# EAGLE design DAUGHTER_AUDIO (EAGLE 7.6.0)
DAUGHTER CARD AUDIO

## Sheet 1 of 3: HDK INTERFACE
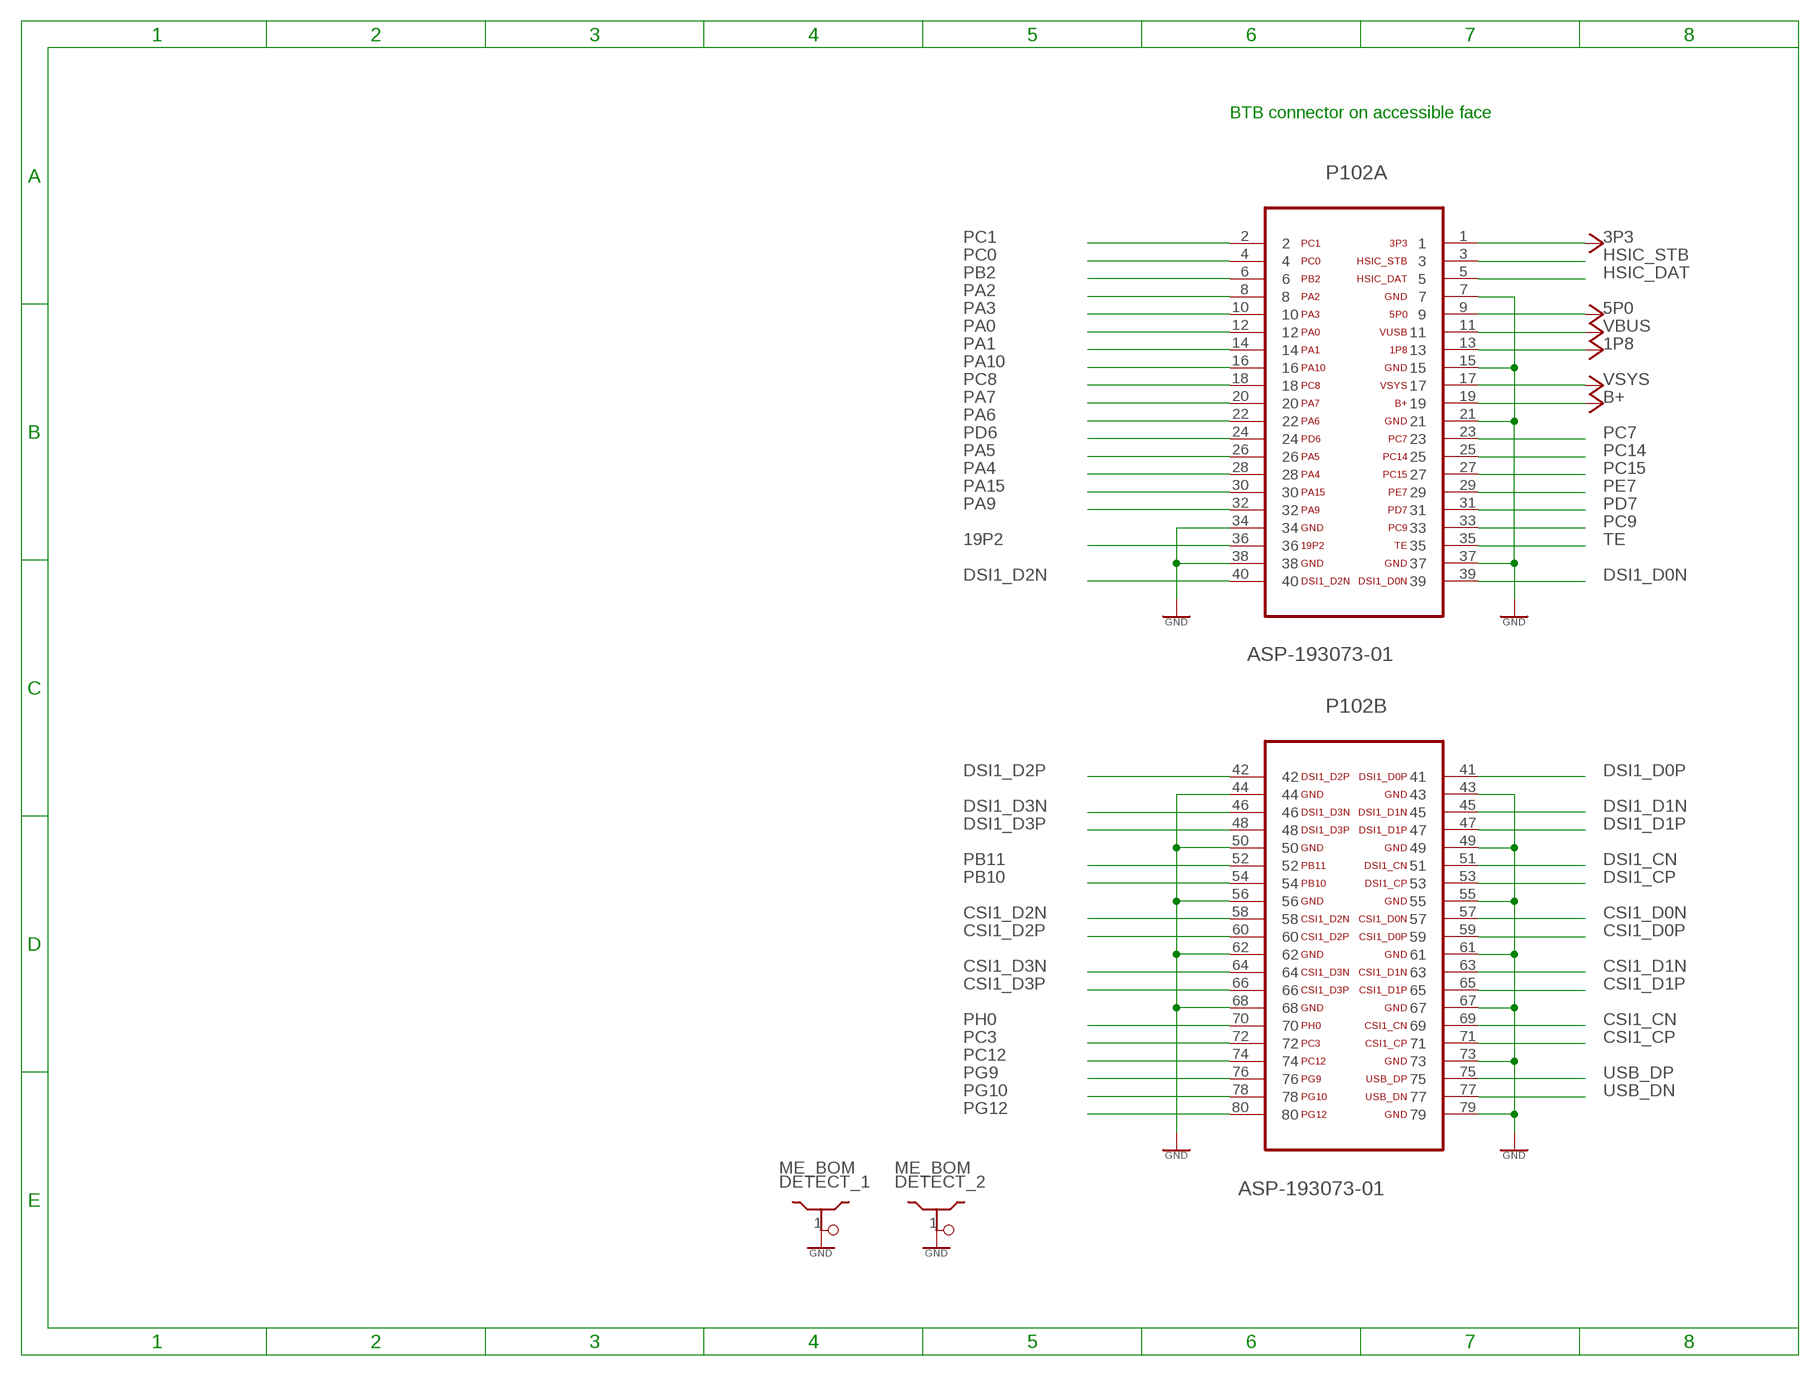
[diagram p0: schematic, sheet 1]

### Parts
DETECT_1  ME_BOM  SHIELDDETECT  [PLUG]
DETECT_2  ME_BOM  SHIELDDETECT  [PLUG]
P102  ASP-193073-01  FTMH-140-02-L-DV-ES-P-TR  [FTMH-140-02-L-DV-ES-P-TR]

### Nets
1P8: P102.13 ; also sheet 2,3
3P3: P102.1 ; also sheet 2
5P0: P102.9
19P2: P102.36
B+: P102.19 ; also sheet 3
CSI1_CN: P102.69
CSI1_CP: P102.71
CSI1_D0N: P102.57
CSI1_D0P: P102.59
CSI1_D1N: P102.63
CSI1_D1P: P102.65
CSI1_D2N: P102.58
CSI1_D2P: P102.60
CSI1_D3N: P102.64
CSI1_D3P: P102.66
DSI1_CN: P102.51
DSI1_CP: P102.53
DSI1_D0N: P102.39
DSI1_D0P: P102.41
DSI1_D1N: P102.45
DSI1_D1P: P102.47
DSI1_D2N: P102.40
DSI1_D2P: P102.42
DSI1_D3N: P102.46
DSI1_D3P: P102.48
GND: DETECT_1.1 DETECT_2.1 P102.7 P102.15 P102.21 P102.34 P102.37 P102.38 P102.43 P102.44 P102.49 P102.50 P102.55 P102.56 P102.61 P102.62 P102.67 P102.68 P102.73 P102.79 ; also sheet 2,3
HSIC_DAT: P102.5
HSIC_STB: P102.3
PA0: P102.12
PA1: P102.14
PA2: P102.8
PA3: P102.10
PA4: P102.28
PA5: P102.26
PA6: P102.22
PA7: P102.20
PA9: P102.32
PA10: P102.16
PA15: P102.30
PB2: P102.6
PB10: P102.54 ; also sheet 2
PB11: P102.52 ; also sheet 2
PC0: P102.4 ; also sheet 3
PC1: P102.2 ; also sheet 3
PC3: P102.72
PC7: P102.23 ; also sheet 3
PC8: P102.18
PC9: P102.33
PC12: P102.74
PC14: P102.25 ; also sheet 3
PC15: P102.27 ; also sheet 3
PD6: P102.24
PD7: P102.31 ; also sheet 3
PE7: P102.29 ; also sheet 3
PG9: P102.76 ; also sheet 2
PG10: P102.78 ; also sheet 3
PG12: P102.80
PH0: P102.70 ; also sheet 3
TE: P102.35
USB_DN: P102.77
USB_DP: P102.75
VBUS: P102.11
VSYS: P102.17

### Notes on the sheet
- BTB connector on accessible face

## Sheet 2 of 3: Identification
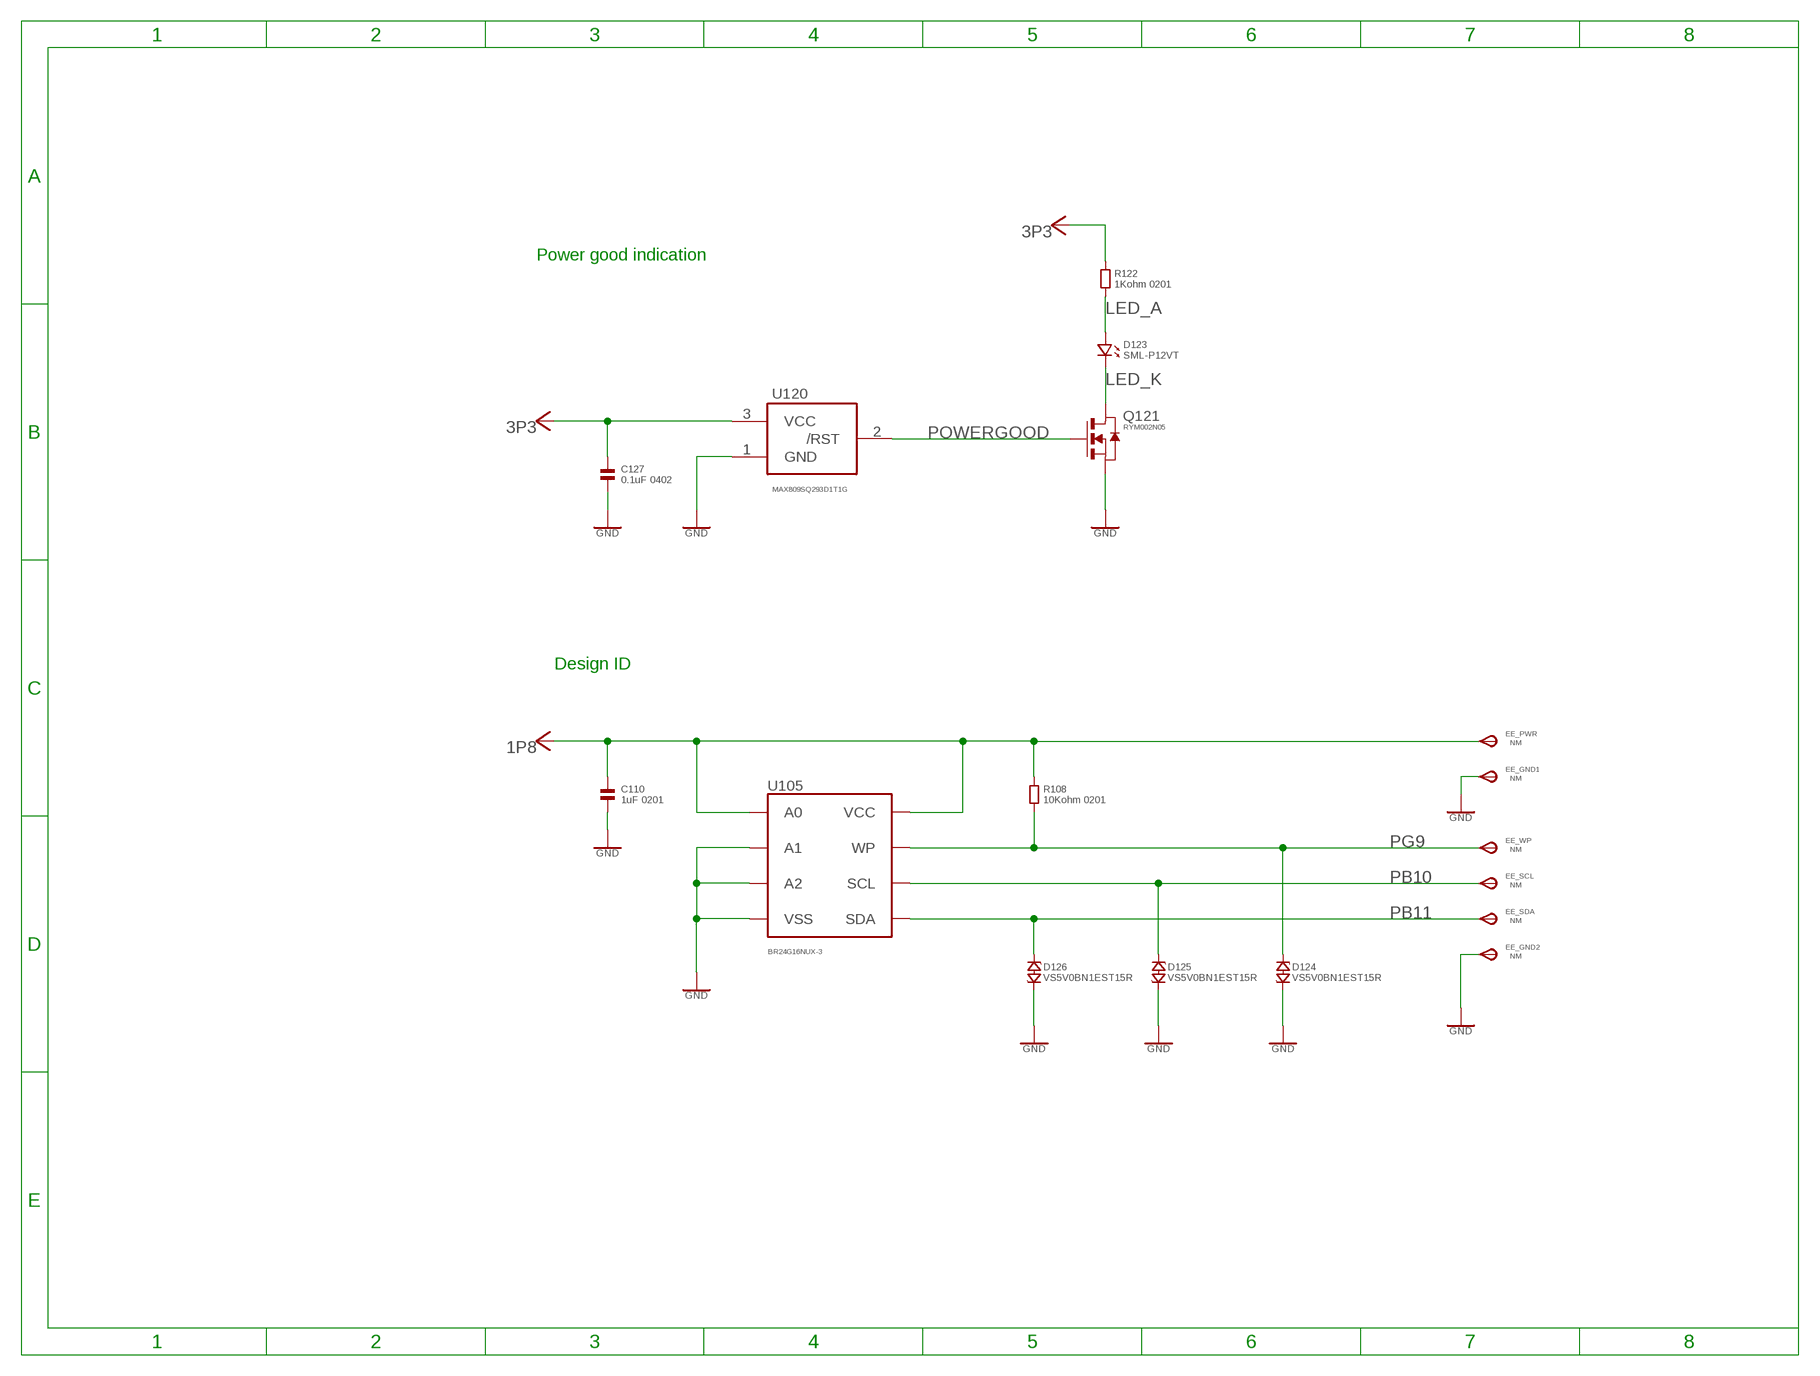
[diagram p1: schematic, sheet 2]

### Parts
C110  1uF 0201  CAPACITOR.0201  [0201]
C127  0.1uF 0402  CAPACITOR.0402  [0402]
D123  SML-P12VT  LED.0503  [0503.LED]
D124  VS5V0BN1EST15R  ESD_VARISTOR.0201  [CHIP_0201]
D125  VS5V0BN1EST15R  ESD_VARISTOR.0201  [CHIP_0201]
D126  VS5V0BN1EST15R  ESD_VARISTOR.0201  [CHIP_0201]
EE_GND1  NM  TPSTP11R  [TP11R]
EE_GND2  NM  TPSTP11R  [TP11R]
EE_PWR  NM  TPSTP11R  [TP11R]
EE_SCL  NM  TPSTP11R  [TP11R]
EE_SDA  NM  TPSTP11R  [TP11R]
EE_WP  NM  TPSTP11R  [TP11R]
Q121  RYM002N05  FET-NRYM002N05  [VMT3]
R108  10Kohm 0201  RESISTOR.0201  [0201]
R122  1Kohm 0201  RESISTOR.0201  [0201]
U105  BR24G16NUX-3  EEPROMDFN8  [DFN-8]
U120  MAX809SQ293D1T1G  MAX809  [SC70-3L]

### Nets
1P8: C110.1 EE_PWR.TP(PP) R108.1 U105.P$1(A0) U105.P$8(VCC) ; also sheet 1,3
3P3: C127.1 R122.1 U120.3(VCC) ; also sheet 1
GND: C110.2 C127.2 D124.P$2 D125.P$2 D126.P$2 EE_GND1.TP(PP) EE_GND2.TP(PP) Q121.2(S) U105.P$2(A1) U105.P$3(A2) U105.P$4(VSS) U105.P$9(VSS) U120.1(GND) ; also sheet 1,3
LED_A: D123.P$1 R122.2
LED_K: D123.P$2 Q121.3(D)
PB10: D125.P$1 EE_SCL.TP(PP) U105.P$6(SCL) ; also sheet 1
PB11: D126.P$1 EE_SDA.TP(PP) U105.P$5(SDA) ; also sheet 1
PG9: D124.P$1 EE_WP.TP(PP) R108.2 U105.P$7(WP) ; also sheet 1
POWERGOOD: Q121.1(G) U120.2(/RST)

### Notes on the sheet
- Power good indication
- Design ID

## Sheet 3 of 3: LOUD SPEAKER
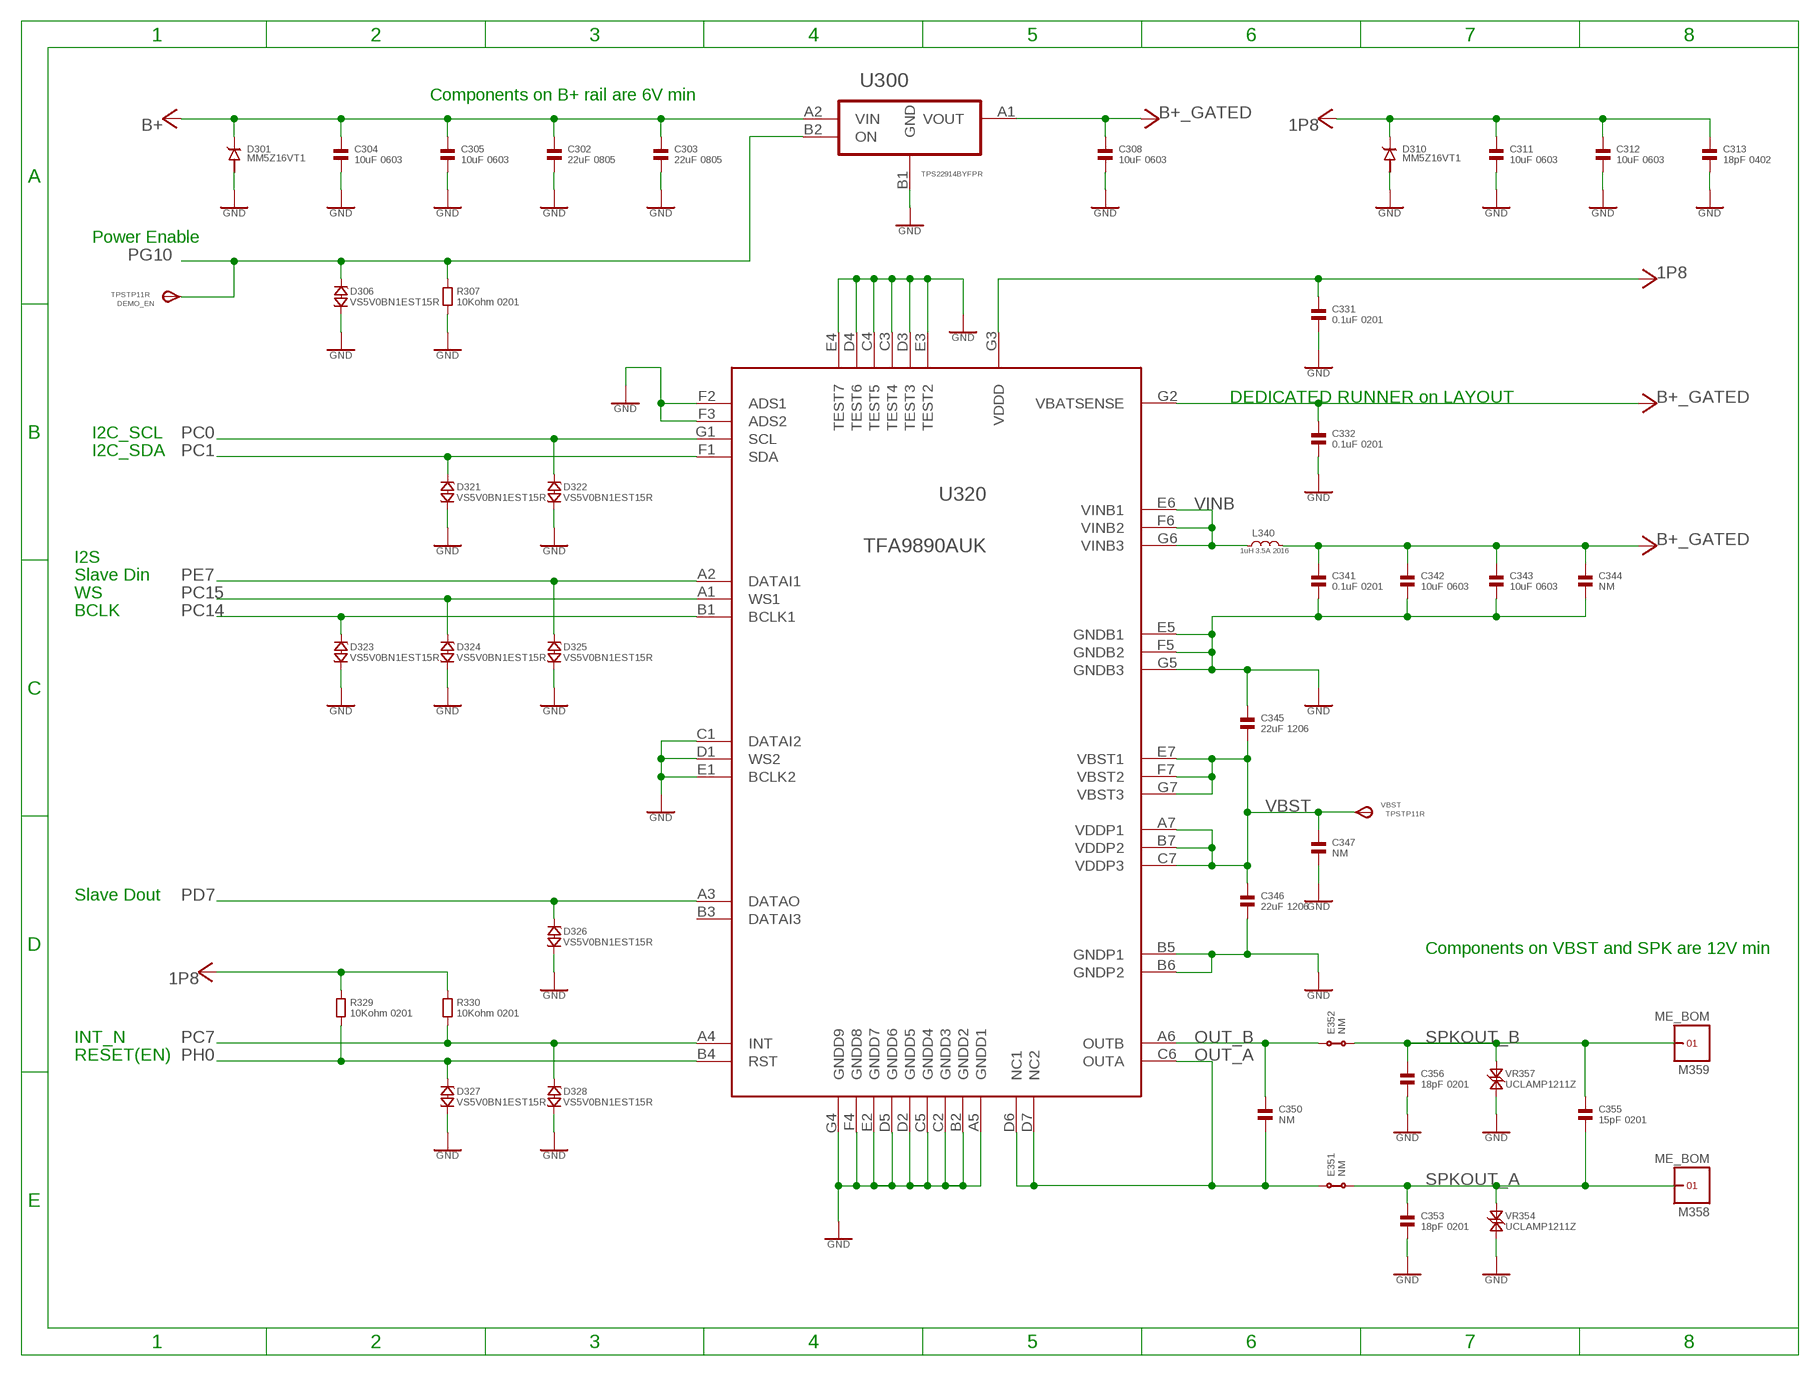
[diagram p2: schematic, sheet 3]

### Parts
C302  22uF 0805  CAPACITOR.0805  [0805]
C303  22uF 0805  CAPACITOR.0805  [0805]
C304  10uF 0603  CAPACITOR.0603  [0603]
C305  10uF 0603  CAPACITOR.0603  [0603]
C308  10uF 0603  CAPACITOR.0603  [0603]
C311  10uF 0603  CAPACITOR.0603  [0603]
C312  10uF 0603  CAPACITOR.0603  [0603]
C313  18pF 0402  CAPACITOR.0402  [0402]
C331  0.1uF 0201  CAPACITOR.0201  [0201]
C332  0.1uF 0201  CAPACITOR.0201  [0201]
C341  0.1uF 0201  CAPACITOR.0201  [0201]
C342  10uF 0603  CAPACITOR.0603  [0603]
C343  10uF 0603  CAPACITOR.0603  [0603]
C344  NM  CAPACITOR.0402  [0402]
C345  22uF 1206  CAPACITOR.1206  [1206]
C346  22uF 1206  CAPACITOR.1206  [1206]
C347  NM  CAPACITOR.0402  [0402]
C350  NM  CAPACITOR.0201  [0201]
C353  18pF 0201  CAPACITOR.0201  [0201]
C355  15pF 0201  CAPACITOR.0201  [0201]
C356  18pF 0201  CAPACITOR.0201  [0201]
D301  MM5Z16VT1  DIODE.SOD523  [SOD523]
D306  VS5V0BN1EST15R  ESD_VARISTOR.0201  [CHIP_0201]
D310  MM5Z16VT1  DIODE.SOD523  [SOD523]
D321  VS5V0BN1EST15R  ESD_VARISTOR.0201  [CHIP_0201]
D322  VS5V0BN1EST15R  ESD_VARISTOR.0201  [CHIP_0201]
D323  VS5V0BN1EST15R  ESD_VARISTOR.0201  [CHIP_0201]
D324  VS5V0BN1EST15R  ESD_VARISTOR.0201  [CHIP_0201]
D325  VS5V0BN1EST15R  ESD_VARISTOR.0201  [CHIP_0201]
D326  VS5V0BN1EST15R  ESD_VARISTOR.0201  [CHIP_0201]
D327  VS5V0BN1EST15R  ESD_VARISTOR.0201  [CHIP_0201]
D328  VS5V0BN1EST15R  ESD_VARISTOR.0201  [CHIP_0201]
DEMO_EN  TPSTP11R  [TP11R]
E351  NM  SHORT_BAR.0603  [0603_SHORT]
E352  NM  SHORT_BAR.0603  [0603_SHORT]
L340  1uH 3.5A 2016  POWER-INDUCTOR.2016  [2016]
M358  ME_BOM  PUCK.PUCK  [PUCK]
M359  ME_BOM  PUCK.PUCK  [PUCK]
R307  10Kohm 0201  RESISTOR.0201  [0201]
R329  10Kohm 0201  RESISTOR.0201  [0201]
R330  10Kohm 0201  RESISTOR.0201  [0201]
U300  TPS22914BYFPR  [BGA0_75SQ_PS0_4_P4]
U320  TFA9890AUK  [BGA7X7]
VBST  TPSTP11R  [TP11R]
VR354  UCLAMP1211Z  ESD_TVS.0201  [CHIP_0201]
VR357  UCLAMP1211Z  ESD_TVS.0201  [CHIP_0201]

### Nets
1P8: C311.1 C312.1 C313.1 C331.1 D310.1 R329.1 R330.1 U320.G3(VDDD) ; also sheet 1,2
B+: C302.1 C303.1 C304.1 C305.1 D301.1 U300.A2(VIN) ; also sheet 1
B+_GATED: C308.1 C332.1 C341.1 C342.1 C343.1 C344.1 L340.2 U300.A1(VOUT) U320.G2(VBATSENSE)
GND: C302.2 C303.2 C304.2 C305.2 C308.2 C311.2 C312.2 C313.2 C331.2 C332.2 C341.2 C342.2 C343.2 C344.2 C345.1 C346.2 C347.2 C353.2 C356.2 D301.2 D306.P$2 D310.2 D321.P$2 D322.P$2 D323.P$2 D324.P$2 D325.P$2 D326.P$2 D327.P$2 D328.P$2 R307.2 U300.B1(GND) U320.A5(GNDD1) U320.B2(GNDD2) U320.B5(GNDP1) U320.B6(GNDP2) U320.C1(DATAI2) U320.C2(GNDD3) U320.C3(TEST4) U320.C4(TEST5) U320.C5(GNDD4) U320.D1(WS2) U320.D2(GNDD5) U320.D3(TEST3) U320.D4(TEST6) U320.D5(GNDD6) U320.E1(BCLK2) U320.E2(GNDD7) U320.E3(TEST2) U320.E4(TEST7) U320.E5(GNDB1) U320.F2(ADS1) U320.F3(ADS2) U320.F4(GNDD8) U320.F5(GNDB2) U320.G4(GNDD9) U320.G5(GNDB3) VR354.P$2 VR357.P$2 ; also sheet 1,2
OUT_A: C350.2 E351.1 U320.C6(OUTA) U320.D6(NC1) U320.D7(NC2)
OUT_B: C350.1 E352.1 U320.A6(OUTB)
PC0: D322.P$1 U320.G1(SCL) ; also sheet 1
PC1: D321.P$1 U320.F1(SDA) ; also sheet 1
PC7: D328.P$1 R330.2 U320.A4(INT) ; also sheet 1
PC14: D323.P$1 U320.B1(BCLK1) ; also sheet 1
PC15: D324.P$1 U320.A1(WS1) ; also sheet 1
PD7: D326.P$1 U320.A3(DATAO) ; also sheet 1
PE7: D325.P$1 U320.A2(DATAI1) ; also sheet 1
PG10: D306.P$1 DEMO_EN.TP(PP) R307.1 U300.B2(ON) ; also sheet 1
PH0: D327.P$1 R329.2 U320.B4(RST) ; also sheet 1
SPKOUT_A: C353.1 C355.2 E351.2 M358.1 VR354.P$1
SPKOUT_B: C355.1 C356.1 E352.2 M359.1 VR357.P$1
VBST: C345.2 C346.1 C347.1 U320.A7(VDDP1) U320.B7(VDDP2) U320.C7(VDDP3) U320.E7(VBST1) U320.F7(VBST2) U320.G7(VBST3) VBST.TP(PP)
VINB: L340.1 U320.E6(VINB1) U320.F6(VINB2) U320.G6(VINB3)
Unconnected: U320.B3(DATAI3)

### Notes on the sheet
- Components on B+ rail are 6V min
- Power Enable
- DEDICATED RUNNER on LAYOUT
- I2C_SCL
- I2C_SDA
- I2S
- Slave Din
- WS
- BCLK
- Slave Dout
- Components on VBST and SPK are 12V min
- INT_N
- RESET(EN)

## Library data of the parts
C110 C127 C302-C305 C308 C311-C313 C331 C332 C341-C347 C350 C353 C355 C356 = MOTO_LIB:CAPACITOR: Ceramic Capacitor, Generic
D123 = MOTO_LIB:LED: LED GENERIC, single, 2 pin; MPN: SML-P12VT; SUPPLIER: ROHM
D124-D126 D306 D321-D328 = MOTO_LIB:ESD_VARISTOR: GENERIC varistor,single, 2 pin; MPN: VS5V0BN1EST15R; SUPPLIER: ROHM
D301 D310 = MOTO_LIB:DIODE: DIODE GENERIC, single, 2 pin; MPN: MM5Z16VT1; SUPPLIER: ON_SEMI
DEMO_EN EE_GND1 EE_GND2 EE_PWR EE_SCL EE_SDA EE_WP VBST = MOTO_LIB:TPS: TEST Point, 1mm diameter, gold
DETECT_1 DETECT_2 = MOTO_LIB:SHIELD: Shield, Custom; MPN: refer to ME BOM; SUPPLIER: ref to ME BOM
E351 E352 = MOTO_LIB:SHORT_BAR: SHORT BAR - layout feature
L340 = MOTO_LIB:POWER-INDUCTOR: Inductor, Power
M358 M359 = MOTO_LIB:PUCK: test pad; MPN: refer to ME BOM; SUPPLIER: refer to ME BOM
P102 = MOTO_LIB:FTMH-140-02-L-DV-ES-P-TR: MICRO SOCKET, 1.0MM, SMD, 2X40WAY, MALE; MPN: ASP-193073-01; SUPPLIER: SAMTEC
Q121 = MOTO_LIB:FET-N: Generic NMOS FET; MPN: RYM002N05; SUPPLIER: ROHM
R108 R122 R307 R329 R330 = MOTO_LIB:RESISTOR: Resistor - Generic
U105 = MOTO_LIB:EEPROM: I2C EE PROM, 8 pin; MPN: BR24G16NUX-3; SUPPLIER: ROHM
U120 = MOTO_LIB:MAX809: 3-Pin Microprocessor Reset Circuit; MPN: MAX809SQ293D1T1; SUPPLIER: ON-SEMI
U300 = MOTO_LIB:TPS22914BYFPR: 5V load switch; MPN: TPS22914BYFPR; SUPPLIER: TI
U320 = MOTO_LIB:TFA9890AUK: Audio Power amplifier; MPN: TFA9890AUK; SUPPLIER: NXP
VR354 VR357 = MOTO_LIB:ESD_TVS: GENERIC TVS,single, 2 pin; MPN: UCLAMP1211Z; SUPPLIER: SEMTECH

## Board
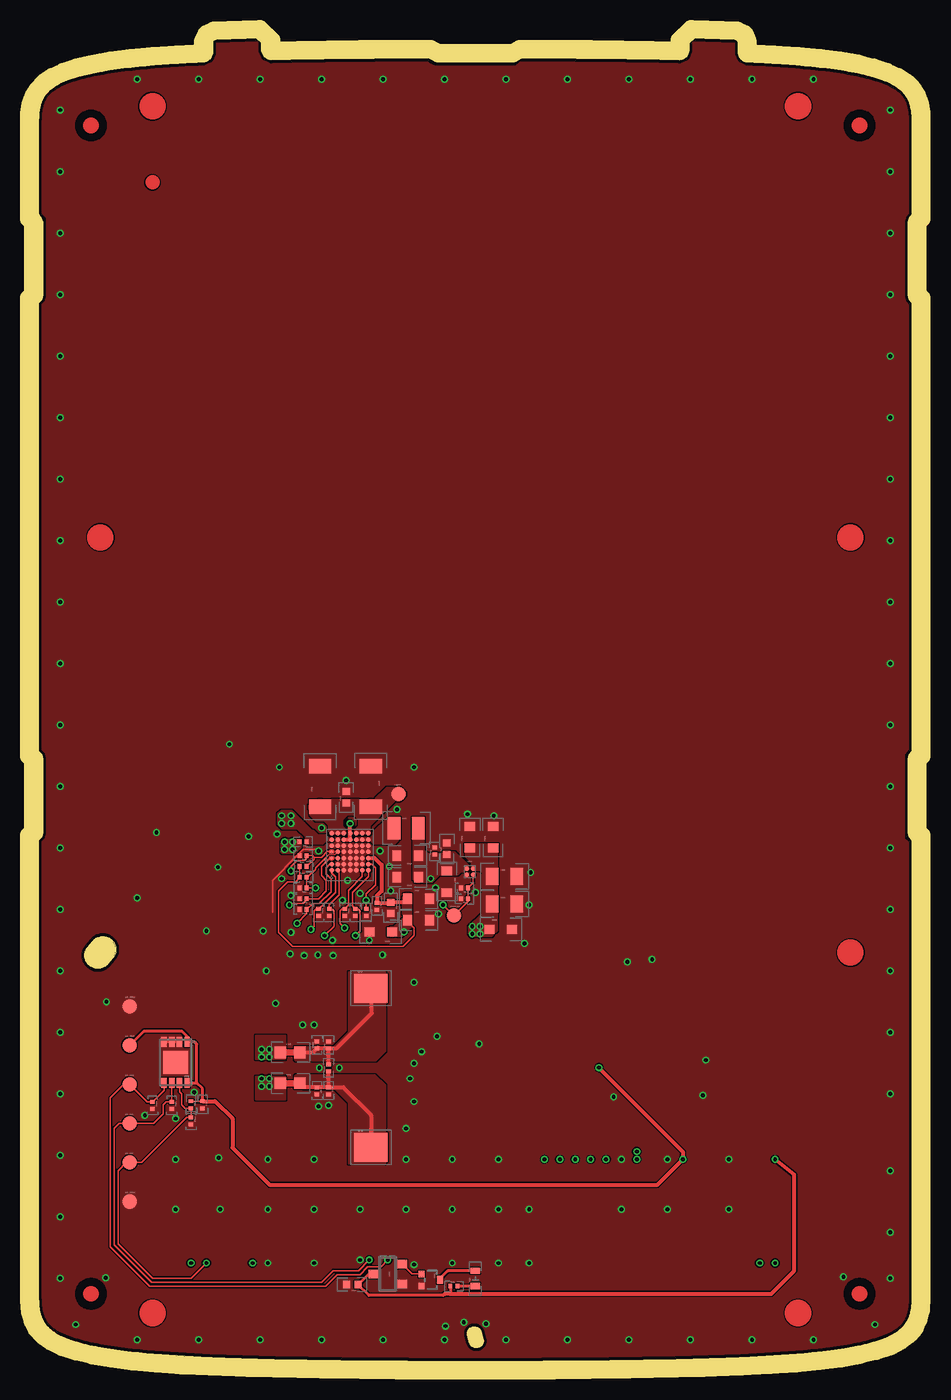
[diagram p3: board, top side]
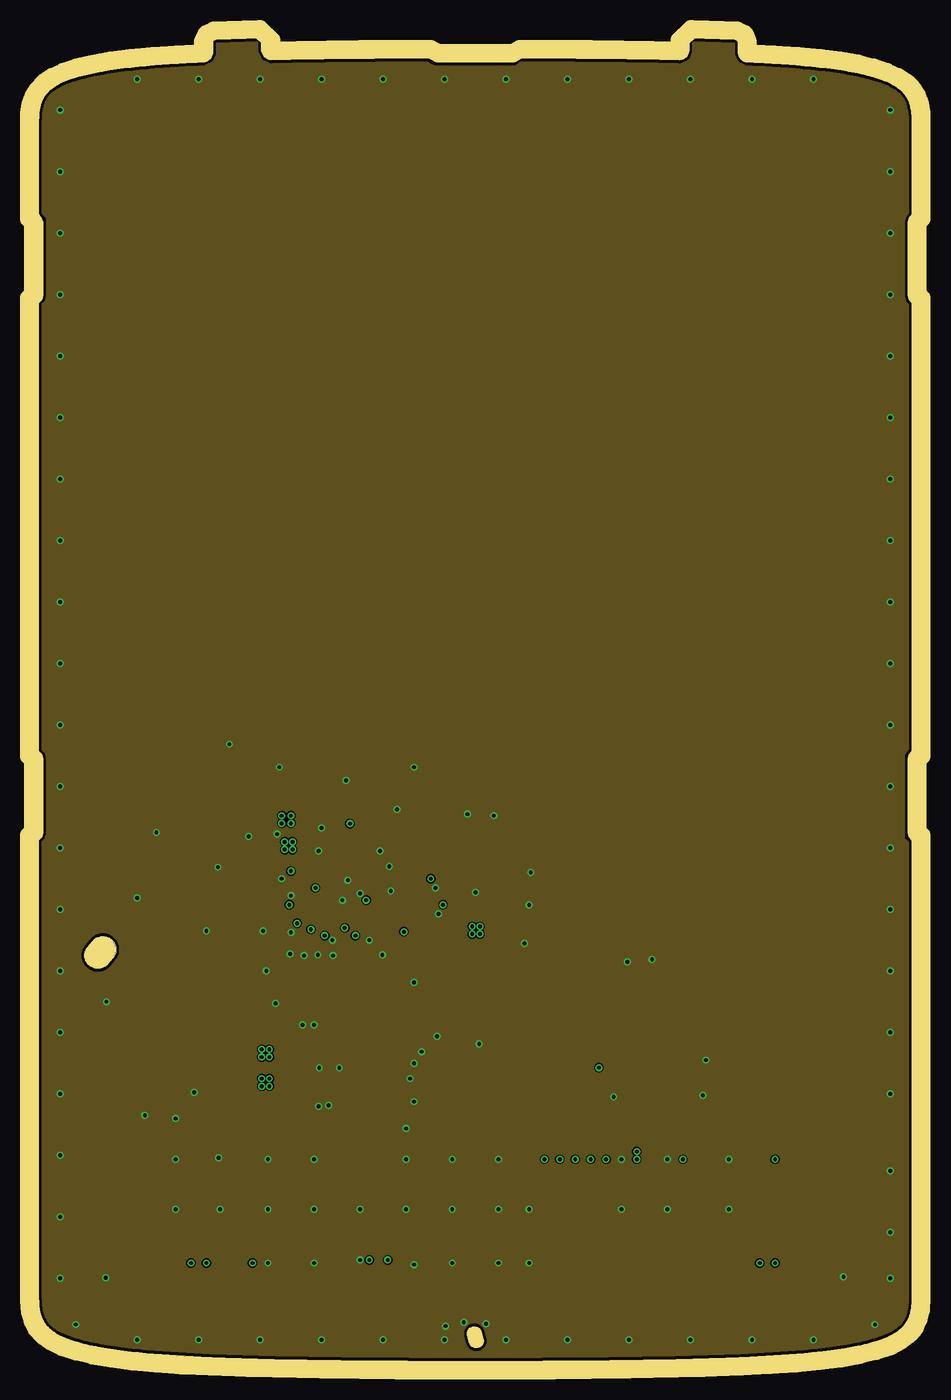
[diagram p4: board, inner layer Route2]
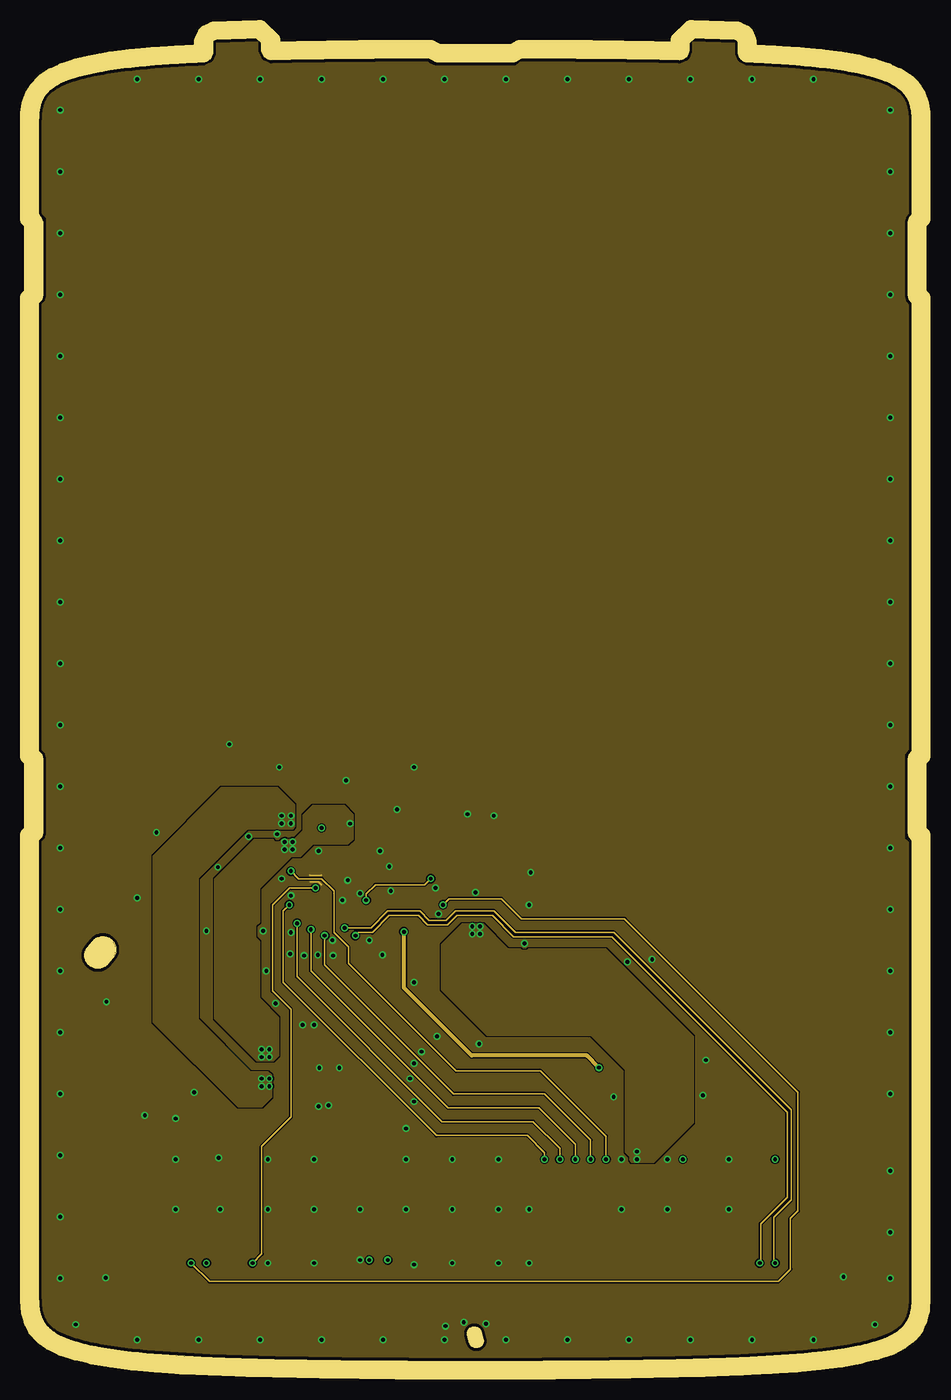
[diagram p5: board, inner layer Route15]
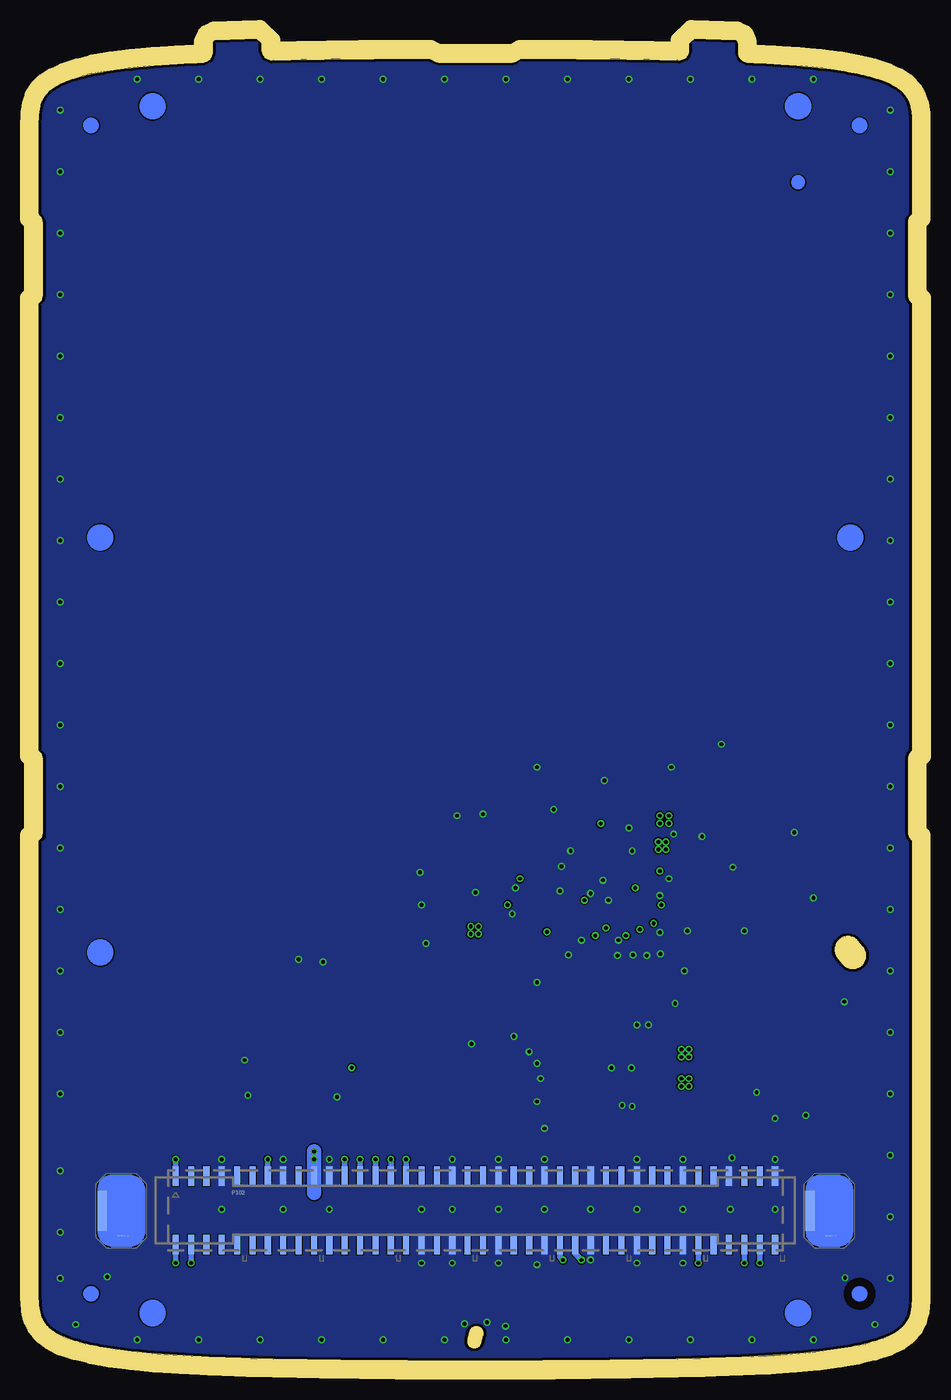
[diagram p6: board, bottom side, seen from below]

Size 56.85 x 86.03 mm. Coordinates in mm from the lower left corner, seen from the top.
Outline: 357 segments
Copper layers (1*2*15*16): Top 0.02mm / dielectric 0.045mm / Route2 0.016mm / dielectric 0.711mm / Route15 0.016mm / dielectric 0.045mm / Bottom 0.02mm
Design rules "constraint": minimum track width 0.08mm, minimum drill 0.25mm, track to track 0.08mm, track to pad 0.08mm, pad to pad 0.08mm, via to via 0.08mm, smd to smd 0.08mm, copper to edge 0.2mm, drill to drill 0.2mm, minimum pad ring 0.1mm, minimum via ring 0.1mm, stop-mask expansion 0mil, vias tented up to drill 0.25mm, thermal gap 0mil
tRestrict: area 3.4,3.4 to 4.4,5.4; area 2.4,3.4 to 3.4,5.4; area 53.4,3.4 to 54.4,5.4; area 52.4,3.4 to 53.4,5.4; area 3.4,79.4 to 4.4,81.4; area 2.4,79.4 to 3.4,81.4; area 53.4,79.4 to 54.4,81.4; area 52.4,79.4 to 53.4,81.4
bRestrict: area 2.4,3.4 to 3.4,5.4; area 3.4,3.4 to 4.4,5.4
Milling: 125 lines

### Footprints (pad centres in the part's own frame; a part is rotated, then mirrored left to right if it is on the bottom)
0201 = smd 0.25 x 0.3: 1 -0.23,0; 2 0.23,0
0402 = smd 0.45 x 0.5: 1 -0.37,0; 2 0.37,0
0805 = smd 0.8 x 1.1: 1 -0.8,0; 2 0.8,0
0603 = smd 0.58 x 0.68: 1 -0.71,0; 2 0.71,0
1206 = smd 0.96 x 1.46: 1 -1.32,0; 2 1.32,0
0503.LED = smd 0.4 x 0.6: P$1 -0.495,0; P$2 0.495,0
CHIP_0201 = smd 0.25 x 0.3: P$1 -0.23,0; P$2 0.23,0
SOD523 = smd 0.64 x 0.59: 1 -0.73,0; 2 0.73,0
TP11R = smd 0.95 x 0.95: TP 0,0
PLUG = smd 0.6 x 2.6: 1 -1.25,0
0603_SHORT = smd 0.76 x 0.76: 1 -0.63,0; 2 0.63,0
2016 = smd 0.82 x 1.46: 1 -0.79,0; 2 0.79,0
PUCK = smd 2.2 x 1.9: 1 0,0
FTMH-140-02-L-DV-ES-P-TR = smd 0.4 x 1.263: 1 -19.5,2.223; 2 -19.5,-2.223; 3 -18.5,2.223; 4 -18.5,-2.223; 5 -17.5,2.223; 6 -17.5,-2.223; 7 -16.5,2.223; 8 -16.5,-2.223; 9 -15.5,2.223; 10 -15.5,-2.223; 11 -14.5,2.223; 12 -14.5,-2.223; 13 -13.5,2.223; 14 -13.5,-2.223; 15 -12.5,2.223; 16 -12.5,-2.223; 17 -11.5,2.223; 18 -11.5,-2.223; 19 -10.5,2.223; 20 -10.5,-2.223; 21 -9.5,2.223; 22 -9.5,-2.223; 23 -8.5,2.223; 24 -8.5,-2.223; 25 -7.5,2.223; 26 -7.5,-2.223; 27 -6.5,2.223; 28 -6.5,-2.223; 29 -5.5,2.223; 30 -5.5,-2.223; 31 -4.5,2.223; 32 -4.5,-2.223; 33 -3.5,2.223; 34 -3.5,-2.223; 35 -2.5,2.223; 36 -2.5,-2.223; 37 -1.5,2.223; 38 -1.5,-2.223; 39 -0.5,2.223; 40 -0.5,-2.223; 41 0.5,2.223; 42 0.5,-2.223; 43 1.5,2.223; 44 1.5,-2.223; 45 2.5,2.223; 46 2.5,-2.223; 47 3.5,2.223; 48 3.5,-2.223; 49 4.5,2.223; 50 4.5,-2.223; 51 5.5,2.223; 52 5.5,-2.223; 53 6.5,2.223; 54 6.5,-2.223; 55 7.5,2.223; 56 7.5,-2.223; 57 8.5,2.223; 58 8.5,-2.223; 59 9.5,2.223; 60 9.5,-2.223; 61 10.5,2.223; 62 10.5,-2.223; 63 11.5,2.223; 64 11.5,-2.223; 65 12.5,2.223; 66 12.5,-2.223; 67 13.5,2.223; 68 13.5,-2.223; 69 14.5,2.223; 70 14.5,-2.223; 71 15.5,2.223; 72 15.5,-2.223; 73 16.5,2.223; 74 16.5,-2.223; 75 17.5,2.223; 76 17.5,-2.223; 77 18.5,2.223; 78 18.5,-2.223; 79 19.5,2.223; 80 19.5,-2.223
VMT3 = smd 0.42 x 0.4: 1 -0.4,-0.6; 2 0.4,-0.6 | smd 0.52 x 0.4: 3 0,0.6
DFN-8 = smd 0.35 x 0.65: P$1 -0.75,-1.325; P$2 -0.25,-1.325; P$3 0.25,-1.325; P$4 0.75,-1.325; P$5 0.75,1.325; P$6 0.25,1.325; P$7 -0.25,1.325; P$8 -0.75,1.325 | smd 1.6 x 1.5: P$9 0,0
SC70-3L = smd 0.55 x 0.63: 1 -0.65,-0.94; 3 0,0.94 | smd 0.555 x 0.63: 2 0.65,-0.94
BGA0_75SQ_PS0_4_P4 = smd 0.32 x 0.32: A1 -0.2,0.2; A2 0.2,0.2; B1 -0.2,-0.2; B2 0.2,-0.2
BGA7X7 = smd 0.32 x 0.32: A1 -1,1.2; A2 -0.6,1.2; A5 0.6,1.2; A6 1,1.2; A7 1.4,1.2; B1 -1,0.8; B2 -0.6,0.8; B3 -0.2,0.8; B4 0.2,0.8; B5 0.6,0.8; B6 1,0.8; B7 1.4,0.8; C1 -1,0.4; C2 -0.6,0.4; C3 -0.2,0.4; C4 0.2,0.4; C5 0.6,0.4; C6 1,0.4; C7 1.4,0.4; D1 -1,0; D2 -0.6,0; D3 -0.2,0; D4 0.2,0; D5 0.6,0; D6 1,0; D7 1.4,0; E1 -1,-0.4; E2 -0.6,-0.4; E3 -0.2,-0.4; E4 0.2,-0.4; E5 0.6,-0.4; E6 1,-0.4; E7 1.4,-0.4; F1 -1,-0.8; F2 -0.6,-0.8; F3 -0.2,-0.8; F4 0.2,-0.8; F5 0.6,-0.8; F6 1,-0.8; F7 1.4,-0.8; G1 -1,-1.2; G2 -0.6,-1.2; G3 -0.2,-1.2; G4 0.2,-1.2; G5 0.6,-1.2; G6 1,-1.2; G7 1.4,-1.2 | smd 0.22 x 0.22: A3 -0.2,1.2; A4 0.2,1.2

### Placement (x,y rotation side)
C110  10.67,16.67 270 top
C127  20.42,4.97 180 top
C302  30.32,31.52 0 top
C303  30.32,29.72 0 top
C304  28.07,34.07 90 top
C305  29.57,34.07 90 top
C308  26.57,31.17 270 top
C311  24.72,28.67 0 top
C312  24.72,30.07 0 top
C313  22.92,29.47 270 top
C331  22.02,29.57 270 top
C332  21.32,29.17 270 top
C341  25.77,33.17 90 top
C342  24.02,32.87 180 top
C343  24.02,31.47 180 top
C344  26.57,33.32 90 top
C345  21.62,37.37 270 top
C346  18.32,37.37 90 top
C347  20.02,36.67 90 top
C350  17.22,33.77 180 top
C353  18.87,20.57 90 top
C355  18.87,19.07 90 top
C356  18.87,17.57 270 top
D123  28.42,5.37 90 top
D124  9.92,15.62 270 top
D125  8.67,16.62 270 top
D126  7.42,16.62 270 top
D301  30.07,28.07 0 top
D306  27.72,30.77 180 top
D310  22.27,27.92 180 top
D321  19.92,29.17 270 top
D322  20.62,29.17 270 top
D323  18.92,29.17 270 top
D324  18.22,29.17 270 top
D325  17.22,29.37 180 top
D326  17.22,30.07 180 top
D327  17.22,30.77 180 top
D328  17.22,32.87 180 top
DEMO_EN  27.02,28.97 0 top
DETECT_1  51.45,9.77 0 bottom
DETECT_2  5.39,9.77 0 bottom
E351  16.37,20.07 0 top
E352  16.37,18.07 0 top
EE_GND1  5.92,10.37 0 top
EE_GND2  5.92,23.07 0 top
EE_PWR  5.92,20.53 0 top
EE_SCL  5.92,15.45 0 top
EE_SDA  5.92,17.99 0 top
EE_WP  5.92,12.91 0 top
L340  23.92,34.67 0 top
M358  21.62,24.25 0 top
M359  21.62,13.9 0 top
P102  28.42,9.8 0 bottom
Q121  25.52,5.27 270 top
R108  9.92,16.67 270 top
R122  27.02,4.87 0 top
R307  27.72,30.07 180 top
R329  17.22,31.47 0 top
R330  17.22,32.17 0 top
U105  8.92,19.42 180 top
U120  22.72,5.67 90 top
U300  28.07,31.82 0 top
U320  20.27,32.92 90 top
VBST  23.42,36.87 0 top
VR354  18.12,20.57 90 top
VR357  18.12,17.57 270 top

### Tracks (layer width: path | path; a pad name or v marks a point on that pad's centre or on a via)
1P8  (via drill 0.25)
  Top 0.1: R108.1 C110.1 | R330.1 R329.1 16.99,31.44 16.72,31.17 16.22,31.17 15.62,30.57 15.62,27.87 16.52,26.97 23.72,26.97 24.42,27.67 24.42,28.17 24.22,28.37 24.22,28.46 C311.1 | U320.G3
  Top 0.2: EE_PWR.TP 6.86,21.47 9.32,21.47 9.67,21.12 U105.P$1 10.15,20.75 10.3,20.6 10.3,18.1 | U105.P$8 10.3,18.1 | 10.3,18.1 10.67,17.72 C110.1
  Top 0.25: U320.G3 21.86,32.73 22.32,32.27 22.32,30.57 22.02,30.27 C331.1 22.88,29.8 C313.1 23.78,29.84 C312.1 | C110.1 11.49,16.9 12.62,15.77 12.62,13.87 15.02,11.47 40.27,11.47 v41.92,13.12 41.92,13.62 v36.46,19.08
  Route15 0.25: v36.46,19.08 35.67,19.87 28.17,19.87 23.77,24.27 v23.77,27.92
  Bottom 0.35: P102.13 v41.92,13.12
  pour Top: 23.72,30.42 24.17,30.42 24.27,30.32 24.27,28.27 23.62,27.62 22.87,27.62 22.77,27.72 22.77,28.17 22.82,28.22 23.12,28.22 23.67,28.77 23.67,30.37
3P3  (via drill 0.25)
  Top 0.2: U120.3 21.49,5.67 C127.1 21.49,4.27 26.32,4.27 26.42,4.37 | R122.1 26.79,4.37
  Top 0.25: v47.92,13.12 49.17,12.12 49.17,5.87 47.67,4.37 26.79,4.37 26.42,4.37
  Bottom 0.35: P102.1 v47.92,13.12
B+  (via drill 0.25)
  Bottom 0.1: v38.92,13.62 v38.91,13.62 38.91,13.64
  Bottom 0.35: P102.19 v38.92,13.12
  Bottom 0.94: 38.91,10.93 38.91,13.64
  other vias: 28.22,28.27 28.72,28.27 28.72,27.77 28.22,27.77
  pour Route15: 27.57,28.42 28.92,28.42 30.52,26.82 31.32,26.82 31.42,26.72 31.82,26.72 31.92,26.82 36.87,26.82 42.62,21.07 42.62,15.52 40.02,12.92 38.62,12.92 38.47,13.07 38.47,13.32 38.17,13.62 38.17,18.97 35.97,21.17 29.22,21.17 26.22,24.17 26.22,27.07
  pour Top: 27.77,33.62 29.87,33.62 29.87,28.02 29.47,27.62 28.17,27.62 27.97,27.82 27.97,28.22 28.87,29.12 28.87,31.82 28.77,31.92 28.27,31.92 28.17,32.02 28.17,32.42 27.77,32.82
B+_GATED  (via drill 0.25)
  Top 0.1: C332.1 v21.32,29.97 21.32,30.37 21.92,30.97 21.92,32.07 21.66,32.33 21.52,32.33 | U320.G2 21.52,32.33 | U320.G2 21.52,32.32 21.52,32.33
  Route15 0.1: v25.52,31.37 25.12,30.97 21.92,30.97 21.32,30.37 v21.32,29.97
  pour Top: 24.37,35.32 25.07,35.32 25.07,33.22 25.27,33.02 26.27,33.02 26.37,33.12 27.07,33.12 27.97,32.22 27.97,31.97 27.92,31.92 27.72,31.92 27.62,31.82 27.47,31.82 27.27,31.62 26.07,31.62 25.57,31.12 24.57,31.12 24.37,31.32
GND  (via drill 0.25)
  Top 0.1: 15.22,29.17 15.22,31.27 16.82,32.87 D328.P$2 | 16.99,33.04 17.22,33.27 18.12,33.27 v18.22,33.17
  Top 0.2: U105.P$4 U105.P$3 U105.P$2
  Route15 0.1: 17.62,31.62 17.67,31.57 18.37,31.57 18.42,31.62 | 17.67,31.17 18.22,31.17 18.42,30.97
  other vias: 14.42,1.37 10.42,1.37 6.42,1.37 22.42,1.37 18.42,1.37 26.42,1.37 30.42,1.37 34.42,1.37 38.42,1.37 42.42,1.37 46.42,1.37 50.42,1.37 54.42,2.37 55.42,8.37 55.42,5.37 55.42,12.37 55.42,17.37 55.42,21.37 55.42,25.37 55.42,29.37 55.42,33.37 55.42,37.37 55.42,41.37 55.42,45.37 55.42,49.37 55.42,53.37 55.42,57.37 55.42,61.37 55.42,65.37 55.42,69.37 55.42,73.37 55.42,77.37 55.42,81.37 50.42,83.37 46.42,83.37 42.42,83.37 38.42,83.37 34.42,83.37 30.42,83.37 26.42,83.37 22.42,83.37 18.42,83.37 14.42,83.37 10.42,83.37 6.42,83.37 1.42,81.37 1.42,77.37 1.42,73.37 1.42,69.37 1.42,65.37 1.42,61.37 1.42,57.37 1.42,53.37 1.42,49.37 1.42,45.37 1.42,41.37 1.42,37.37 1.42,33.37 1.42,29.37 1.42,25.37 4.42,23.37 1.42,21.37 1.42,17.37 1.42,13.37 1.42,9.37 1.42,5.37 2.42,2.37 8.92,13.12 11.72,13.22 14.92,13.12 17.92,13.12 23.92,13.12 26.92,13.12 29.92,9.87 31.92,9.87 26.92,9.87 23.92,9.87 20.92,9.87 17.92,9.87 14.92,9.87 11.82,9.87 8.92,9.87 8.92,15.77 10.12,17.47 14.92,6.37 17.92,6.37 20.92,6.57 24.42,6.27 26.92,6.37 29.92,6.37 31.92,6.37 44.92,9.87 40.92,9.87 37.92,9.87 37.92,13.12 40.92,13.12 44.92,13.12 6.92,15.97 29.12,2.42 27.67,2.52 26.47,2.27 52.37,5.47 4.37,5.42 29.92,13.12 12.42,40.12 15.67,38.62 20.02,37.77 24.42,38.62 29.62,35.47 27.92,35.57 23.32,35.87 7.67,34.37 6.42,30.12 32.02,31.77 31.92,29.67 31.62,27.17 15.52,34.27 13.67,34.12 11.67,32.12 10.92,27.97 15.82,31.37 14.62,27.97 14.82,25.37 15.42,23.27 17.17,21.87 17.92,21.87 19.17,26.37 18.17,26.42 17.27,26.37 16.37,26.47 16.42,27.87 19.12,27.37 16.42,30.27 28.42,30.47 24.42,24.62 22.37,26.42 21.52,27.37 19.77,29.97 20.92,30.42 20.12,31.27 22.22,33.17 22.82,32.17 22.92,30.57 26.02,29.07 25.82,30.77 18.42,34.67 37.42,17.17 43.22,17.27 43.42,19.57 39.92,26.12 38.32,25.97 28.67,20.62 25.92,21.12 24.92,20.12 24.42,19.37 24.17,18.37 24.42,16.87 23.92,15.12 18.27,19.07 19.57,19.07 18.87,16.62 18.22,16.57
  pour Top (rank 2): 25.82,84.22 31.07,84.22 31.57,84.67 36.72,84.67 41.82,84.57 42.12,84.67 42.32,84.97 42.42,85.17 42.42,85.57 42.72,85.97 45.32,85.87 45.42,85.67 45.42,84.97 45.62,84.57 45.82,84.47 46.12,84.37 47.12,84.37 50.02,84.17 51.72,83.97 53.32,83.67 54.82,83.27 55.72,82.87 56.22,82.47 56.52,82.07 56.72,81.47 56.82,80.77 56.82,74.97 56.42,74.47 56.32,74.07 56.32,69.27 56.42,68.87 56.82,68.47 56.82,39.97 56.32,39.47 56.32,33.97 56.82,33.57 56.82,4.87 56.72,3.47 56.52,2.67 56.12,2.17 55.52,1.77 54.22,1.27 52.92,0.97 51.62,0.77 48.72,0.47 44.72,0.27 43.62,0.27 43.32,0.37 38.32,0.27 38.02,0.17 36.62,0.07 20.12,0.07 18.72,0.17 18.52,0.27 13.52,0.37 13.22,0.27 10.82,0.37 7.02,0.57 3.92,0.97 2.32,1.37 1.32,1.77 0.72,2.17 0.42,2.47 0.22,2.97 0.12,3.47 0.02,4.47 0.02,33.57 0.42,33.97 0.52,34.27 0.52,39.27 0.32,39.67 0.12,39.97 0.02,40.07 0.02,68.47 0.32,68.77 0.52,69.17 0.52,74.37 0.02,74.87 0.02,80.27 0.12,81.27 0.42,82.27 0.72,82.57 1.72,83.17 3.02,83.57 4.52,83.87 7.02,84.17 9.92,84.37 10.82,84.37 11.22,84.57 11.42,84.87 11.42,85.67 11.52,85.87 14.12,85.97 14.42,85.67 14.42,85.07 14.62,84.77 14.92,84.57 15.52,84.57 19.92,84.67 25.17,84.67 25.37,84.42
  pour Bottom (rank 2): 25.82,84.27 31.02,84.27 31.42,84.47 31.62,84.67 36.72,84.67 41.82,84.57 42.12,84.67 42.32,84.97 42.42,85.17 42.42,85.57 42.72,85.97 45.32,85.87 45.42,85.67 45.42,84.97 45.62,84.57 45.82,84.47 46.12,84.37 47.12,84.37 50.02,84.17 51.72,83.97 53.32,83.67 54.82,83.27 55.72,82.87 56.22,82.47 56.52,82.07 56.72,81.47 56.82,80.77 56.82,74.97 56.42,74.47 56.32,74.07 56.32,69.27 56.42,68.87 56.82,68.47 56.82,39.97 56.32,39.47 56.32,33.97 56.82,33.57 56.82,4.87 56.72,3.47 56.52,2.67 56.12,2.17 55.52,1.77 54.22,1.27 52.92,0.97 51.62,0.77 48.72,0.47 44.72,0.27 43.62,0.27 43.32,0.37 38.32,0.27 38.02,0.17 36.62,0.07 20.12,0.07 18.72,0.17 18.52,0.27 13.52,0.37 13.22,0.27 10.82,0.37 7.02,0.57 3.92,0.97 2.32,1.37 1.32,1.77 0.72,2.17 0.42,2.47 0.22,2.97 0.12,3.47 0.02,4.47 0.02,33.57 0.42,33.97 0.52,34.27 0.52,39.27 0.32,39.67 0.12,39.97 0.02,40.07 0.02,68.47 0.32,68.77 0.52,69.17 0.52,74.37 0.02,74.87 0.02,80.27 0.12,81.27 0.42,82.27 0.72,82.57 1.72,83.17 3.02,83.57 4.52,83.87 7.02,84.17 9.92,84.37 10.82,84.37 11.22,84.57 11.42,84.87 11.42,85.67 11.52,85.87 14.12,85.97 14.42,85.67 14.42,85.07 14.62,84.77 14.92,84.57 15.52,84.57 19.92,84.67 25.32,84.67 25.62,84.37
  pour Route15 (rank 2): 25.82,84.22 31.07,84.22 31.57,84.67 36.72,84.67 41.82,84.57 42.12,84.67 42.32,84.97 42.42,85.17 42.42,85.57 42.72,85.97 45.32,85.87 45.42,85.67 45.42,84.97 45.62,84.57 45.82,84.47 46.12,84.37 47.12,84.37 50.02,84.17 51.72,83.97 53.32,83.67 54.82,83.27 55.72,82.87 56.22,82.47 56.52,82.07 56.72,81.47 56.82,80.77 56.82,74.97 56.42,74.47 56.32,74.07 56.32,69.27 56.42,68.87 56.82,68.47 56.82,39.97 56.32,39.47 56.32,33.97 56.82,33.57 56.82,4.87 56.72,3.47 56.52,2.67 56.12,2.17 55.52,1.77 54.22,1.27 52.92,0.97 51.62,0.77 48.72,0.47 44.72,0.27 43.62,0.27 43.32,0.37 38.32,0.27 38.02,0.17 36.62,0.07 20.12,0.07 18.72,0.17 18.52,0.27 13.52,0.37 13.22,0.27 10.82,0.37 7.02,0.57 3.92,0.97 2.32,1.37 1.32,1.77 0.72,2.17 0.42,2.47 0.22,2.97 0.12,3.47 0.02,4.47 0.02,33.57 0.42,33.97 0.52,34.27 0.52,39.27 0.32,39.67 0.12,39.97 0.02,40.07 0.02,68.47 0.32,68.77 0.52,69.17 0.52,74.37 0.02,74.87 0.02,80.27 0.12,81.27 0.42,82.27 0.72,82.57 1.72,83.17 3.02,83.57 4.52,83.87 7.02,84.17 9.92,84.37 10.82,84.37 11.22,84.57 11.42,84.87 11.42,85.67 11.52,85.87 14.12,85.97 14.42,85.67 14.42,85.07 14.62,84.77 14.92,84.57 15.52,84.57 19.92,84.67 25.17,84.67 25.37,84.42
  pour Route2 (rank 2): 25.82,84.22 31.07,84.22 31.57,84.67 36.72,84.67 41.82,84.57 42.12,84.67 42.32,84.97 42.42,85.17 42.42,85.57 42.72,85.97 45.32,85.87 45.42,85.67 45.42,84.97 45.62,84.57 45.82,84.47 46.12,84.37 47.12,84.37 50.02,84.17 51.72,83.97 53.32,83.67 54.82,83.27 55.72,82.87 56.22,82.47 56.52,82.07 56.72,81.47 56.82,80.77 56.82,74.97 56.42,74.47 56.32,74.07 56.32,69.27 56.42,68.87 56.82,68.47 56.82,39.97 56.32,39.47 56.32,33.97 56.82,33.57 56.82,4.87 56.72,3.47 56.52,2.67 56.12,2.17 55.52,1.77 54.22,1.27 52.92,0.97 51.62,0.77 48.72,0.47 44.72,0.27 43.62,0.27 43.32,0.37 38.32,0.27 38.02,0.17 36.62,0.07 20.12,0.07 18.72,0.17 18.52,0.27 13.52,0.37 13.22,0.27 10.82,0.37 7.02,0.57 3.92,0.97 2.32,1.37 1.32,1.77 0.72,2.17 0.42,2.47 0.22,2.97 0.12,3.47 0.02,4.47 0.02,33.57 0.42,33.97 0.52,34.27 0.52,39.27 0.32,39.67 0.12,39.97 0.02,40.07 0.02,68.47 0.32,68.77 0.52,69.17 0.52,74.37 0.02,74.87 0.02,80.27 0.12,81.27 0.42,82.27 0.72,82.57 1.72,83.17 3.02,83.57 4.52,83.87 7.02,84.17 9.92,84.37 10.82,84.37 11.22,84.57 11.42,84.87 11.42,85.67 11.52,85.87 14.12,85.97 14.42,85.67 14.42,85.07 14.62,84.77 14.92,84.57 15.52,84.57 19.92,84.67 25.17,84.67 25.37,84.42
LED_A
  Top 0.1: R122.2
  Top 0.2: D123.P$1 R122.2
LED_K
  Top 0.2: D123.P$2 26.62,5.87 26.22,5.47 26.22,5.37 Q121.3
OUT_A  (via drill 0.25)
  Top 0.1: U320.D6 U320.D7
  Top 0.25: U320.C6 U320.D6
  Top 0.251: U320.D6 v20.27,34.96
  other vias: 15.02,20.27 15.02,19.77 14.52,19.77 14.52,20.27 16.02,33.77 16.52,33.77 16.52,33.27 16.02,33.27
  pour Route15: 17.87,36.12 19.87,36.12 20.47,35.52 20.47,33.97 20.12,33.62 17.82,33.62 17.02,32.82 16.42,32.82 14.37,30.77 14.37,28.57 14.12,28.32 14.12,27.52 14.37,27.27 14.37,23.57 15.62,22.32 15.62,19.87 15.27,19.52 14.22,19.52 11.47,22.27 11.47,31.32 14.07,33.92 15.22,33.92 15.37,33.77 15.72,33.77 15.87,33.92 16.67,33.92 17.22,34.47 17.22,35.47
  pour Top: 15.92,33.92 16.97,33.92 17.07,33.82 17.07,33.42 16.82,33.17 16.72,33.17 16.72,33.07 16.67,33.02 15.87,33.02 15.77,33.12 15.77,33.77
  pour Top: 14.12,21.17 16.07,21.17 16.07,19.62 14.12,19.62
OUT_B  (via drill 0.25)
  other vias: 15.02,18.37 14.52,18.37 15.02,17.87 14.52,17.87 16.42,34.97 15.82,34.97 15.82,35.47 16.42,35.47
  pour Route15: 11.92,37.32 15.52,37.32 16.67,36.17 16.67,34.77 16.52,34.62 13.57,34.62 10.37,31.42 10.37,22.22 13.77,18.82 14.92,18.82 15.17,18.57 15.17,17.17 14.52,16.52 13.02,16.52 7.47,22.07 7.47,32.82
  pour Top: 15.82,35.82 16.47,35.82 17.77,34.52 17.87,34.52 18.17,34.22 18.67,34.22 18.87,34.02 19.07,34.02 19.12,33.97 19.12,33.87 19.07,33.82 18.67,33.82 18.47,33.62 17.37,33.62 17.37,34.12 16.87,34.62 15.87,34.62 15.57,34.92 15.57,35.57
  pour Top: 14.12,18.52 16.07,18.52 16.07,16.97 14.12,16.97
PB10  (via drill 0.25)
  Top 0.1: v21.52,6.57 20.82,5.87 19.17,5.87 18.42,5.12 7.37,5.12 4.92,7.57 4.92,15.12 5.25,15.45 EE_SCL.TP 7.5,15.45 8.12,16.07 8.12,16.67 8.3,16.85 D125.P$1 U105.P$6
  Bottom 0.35: P102.54 21.92,6.97 v21.52,6.57
PB11  (via drill 0.25)
  Top 0.1: v22.72,6.57 22.27,6.12 21.42,6.12 20.92,5.62 19.42,5.62 18.67,4.87 7.22,4.87 4.67,7.42 4.67,17.12 5.54,17.99 EE_SDA.TP 7.06,16.85 D126.P$1 8.17,17.6 U105.P$5
  Bottom 0.35: P102.52 22.92,6.77 v22.72,6.57
PC0  (via drill 0.25)
  Top 0.1: v20.62,27.67 20.92,27.97 20.92,29.27 20.79,29.4 D322.P$1 20.42,29.6 20.42,30.47 21.46,31.51 U320.G1 | U320.G1 | U320.G1
  Route15 0.1: v20.62,27.67 20.82,27.87 21.72,27.87 22.82,28.97 24.72,28.97 25.32,28.37 26.62,28.37 27.22,28.97 29.52,28.97 30.91,27.59 37.31,27.59 48.72,16.18 48.72,10.65 47,8.93 47,6.45 v46.92,6.37
  Bottom 0.35: P102.4 v46.92,6.37
PC1  (via drill 0.25)
  Top 0.1: v19.92,28.17 19.62,28.47 19.62,29.27 19.75,29.4 D321.P$1 20.17,29.65 20.17,30.62 21.06,31.51 U320.F1 | U320.F1 | U320.F1
  Route15 0.1: v47.92,6.37 47.84,6.46 47.84,9.35 48.97,10.48 48.97,16.33 37.42,27.87 31.02,27.87 29.62,29.27 27.12,29.27 26.52,28.67 25.42,28.67 24.82,29.27 22.72,29.27 21.62,28.17 v19.92,28.17
  Bottom 0.35: P102.2 v47.92,6.37
PC7  (via drill 0.25)
  Top 0.1: 17.92,32.77 18.42,32.77 18.78,33.13 U320.A4 | 17.92,32.77 17.82,32.87 D328.P$1 17.45,32.7 17.32,32.57 16.82,32.57 16.42,32.17 v16.42,31.87 | 17.92,32.77 17.92,32.62 R330.2
  Route15 0.1: v36.92,13.12 36.92,14.62 32.67,18.87 27.17,18.87 20.17,25.87 20.17,26.92 19.22,27.87 19.22,30.57 18.42,31.37 16.92,31.37 v16.42,31.87
  Bottom 0.35: P102.23 v36.92,13.12
PC14  (via drill 0.25)
  Top 0.1: v18.62,27.67 19.22,28.27 19.22,29.27 19.12,29.37 18.95,29.37 D323.P$1 18.92,29.67 19.56,30.31 19.56,31.83 19.52,31.87 | 19.52,31.87 U320.B1 | U320.B1 | U320.B1 19.52,31.92 19.52,31.87
  Route15 0.1: v18.62,27.67 18.62,25.75 27,17.37 32.92,17.37 35.92,14.37 v35.92,13.12
  Bottom 0.35: v35.92,13.12 P102.25
PC15  (via drill 0.25)
  Top 0.1: v17.72,28.07 17.92,28.27 17.92,29.27 18.05,29.4 D324.P$1 18.39,29.57 18.42,29.57 19.32,30.47 19.32,31.47 19.06,31.73 U320.A1 | U320.A1 | U320.A1
  Route15 0.1: v34.92,13.12 34.92,14.1 32.55,16.47 26.63,16.47 17.72,25.38 v17.72,28.07
  Bottom 0.35: v34.92,13.12 P102.27
PD7  (via drill 0.25)
  Top 0.1: v16.32,29.67 16.42,29.77 17.22,29.77 17.45,30 D326.P$1 18.22,30.07 18.72,30.57 18.72,31.27 18.42,31.57 18.42,32.17 18.98,32.73 U320.A3
  Route15 0.1: v32.92,13.12 32.92,13.56 31.81,14.67 25.88,14.67 15.92,24.63 15.92,29.27 v16.32,29.67
  Bottom 0.35: v32.92,13.12 P102.31
PE7  (via drill 0.25)
  Top 0.1: v16.82,28.47 17.45,29.1 D325.P$1 17.85,29.77 18.27,29.77 19.02,30.52 19.02,31.37 18.72,31.67 18.72,32.07 18.98,32.33 U320.A2
  Route15 0.1: v16.82,28.47 16.82,25.01 26.26,15.57 32.18,15.57 33.92,13.83 v33.92,13.12
  Bottom 0.35: v33.92,13.12 P102.29
PG9  (via drill 0.25)
  Top 0.1: v10.92,6.37 9.92,5.37 7.42,5.37 5.17,7.62 5.17,12.37 5.71,12.91 EE_WP.TP 6.71,12.91 9.65,15.85 D124.P$1 R108.2 9.55,16.44 9.32,16.67 9.32,17.37 9.17,17.52 U105.P$7
  Bottom 0.35: P102.76 v10.92,6.37
PG10  (via drill 0.25)
  Top 0.1: v26.32,29.67 DEMO_EN.TP | DEMO_EN.TP 27,28.95 | DEMO_EN.TP 27.95,29.9 R307.1 D306.P$1 28.27,31.09 U300.B2
  Route15 0.1: v9.92,6.37 11.12,5.17 48.12,5.17 48.92,5.97 48.92,9.27 49.42,9.77 49.42,17.48 38.12,28.77 31.42,28.77 30.12,30.07 26.72,30.07 v26.32,29.67
  Bottom 0.35: P102.78 v9.92,6.37
PH0  (via drill 0.25)
  Top 0.05: 19.26,32.93 18.88,32.93
  Top 0.08: 18.88,32.93 18.72,32.77 | U320.B4 19.26,32.93
  Top 0.1: v18.02,30.77 D327.P$1 R329.2 17.52,31.47 18.02,31.97 18.02,32.08 18.72,32.77 | U320.B4
  Route15 0.1: v18.02,30.77 16.32,30.77 15.22,29.67 15.22,24.07 16.43,22.86 16.43,15.88 14.52,13.97 14.52,6.97 v13.92,6.37
  Bottom 0.35: v13.92,6.37 P102.70
POWERGOOD
  Top 0.1: Q121.1 24.31,5.67 U120.2
SPKOUT_A
  Top 0.1: VR354.P$1 18.14,20.34 18.17,20.37 18.15,20.37 VR354.P$1
  Top 0.25: C355.2 C353.1 | C353.1 19.39,20.34 21.67,22.62 21.67,24.2 M358.1 | C353.1 18.2,20.34 18.17,20.37 17.87,20.07 E351.2
  pour Top: 20.17,25.32 22.57,25.32 22.57,20.17 21.92,19.52 16.77,19.52 16.67,19.62 16.67,20.42 19.22,20.42 20.17,21.37
SPKOUT_B
  Top 0.25: C356.1 C355.1 | C356.1 VR357.P$1 17.24,17.8 16.97,18.07 E352.2 | C356.1 19.83,17.8 21.62,16.01 M359.1
  pour Top: 16.67,17.72 16.67,18.52 16.77,18.62 21.87,18.62 22.57,17.92 22.57,12.82 20.17,12.82 20.17,16.82 19.27,17.72
VBST
  pour Top: 17.57,36.52 21.87,36.52 22.67,37.32 23.62,37.32 23.87,37.07 23.87,36.67 23.62,36.42 23.17,36.42 21.57,34.82 21.57,34.32 21.52,34.27 20.62,34.27 20.57,34.32 20.57,34.52 20.82,34.77 20.82,35.27 20.57,35.52 20.07,35.52 19.77,35.22 19.77,34.77 19.97,34.57 19.97,34.32 19.92,34.27 19.12,34.27 18.87,34.52 18.87,34.87 18.62,35.12 18.07,35.12 17.57,35.62
VINB
  pour Top: 23.47,35.37 23.47,33.92 23.17,33.62 21.82,33.62 21.62,33.82 20.67,33.82 20.62,33.87 20.62,33.97 20.67,34.02 20.77,34.02 20.82,34.07 21.62,34.07 21.77,34.22 21.77,34.37 22.77,35.37
(copper drawn outside any net)
  shapes: Bottom circle x24, Top circle x12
